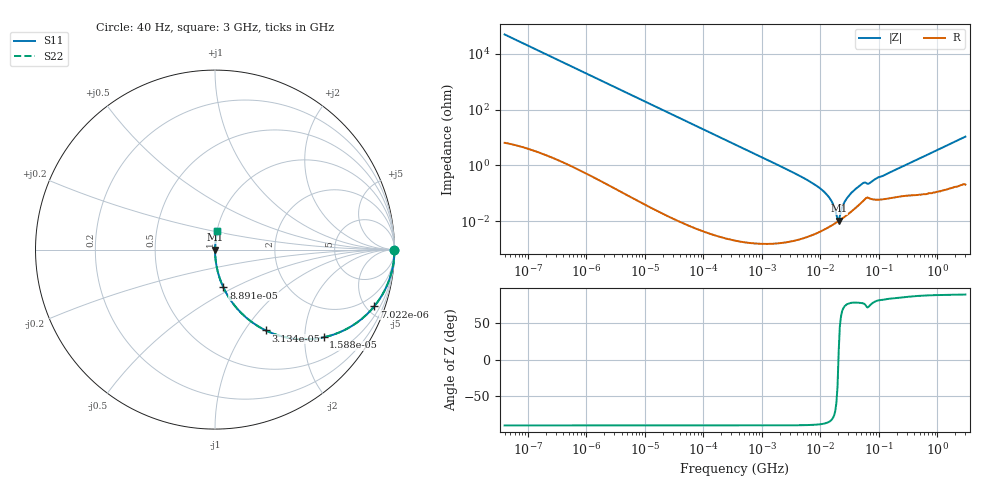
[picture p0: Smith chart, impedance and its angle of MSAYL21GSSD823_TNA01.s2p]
! MSAYL21GSSD823_TNA01  S-PARAMETER MODEL  ( General Type )
! Model Generated by TAIYO YUDEN Corporation (http://www.ty-top.com)
! Version 2.0
! TAIYO YUDEN Control No. 041125
! Copyright(c) 2004 TAIYO YUDEN CO.,LTD. All Rights Reserved.
! Product Description (link to TY-COMPAS)
! https://ds.yuden.co.jp/TYCOMPAS/or/detail?pn=MSAYL21GSSD823KTNA01&u=M
! Products Name : Multilayer Ceramic Capacitors
! Characteristics :
!  Capacitance : 0.082 uF , Rated Voltage : 10V
!  Case Size : 2.0 x 1.25 / 0.079 x 0.049 [mm/inch] , Thickness : 1.25 / 0.049 [mm/inch]
!  (Conditions: Temperature = 25 degC , DC Bias Current/Voltage = 0A / 0V)
! External Node Assignments :
!  1  o---| |---o  2
! GND o---------o GND
! Frequency Range : 40Hz  -  3GHz  [ 401 STEP ]
# MHz S RI R 50
! Freq[MHz].  S11 Real  S11 Imag  S21 Real  S21 Imag  S12 Real  S12 Imag  S22 Real  S22 Imag
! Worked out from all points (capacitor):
!   401 points, 40 Hz to 3 GHz, reference 50 ohm
!   read as one part in series: C = 80.9 nF near 44 Hz
!   lowest |Z| = 10.4 mohm at 20.49 MHz (marker M1)
!   series resonance near 20.3 MHz, so ESL is about 760 pH
!   S11 on the Smith chart (normalised r, x): 40 Hz: open; 7.022 kHz: 1.00, -5.61; 15.88 kHz: 1.00, -2.48; 31.34 kHz: 1.00, -1.26; 88.91 kHz: 1.00, -0.44; 3 GHz: 1.00, +0.22
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4e-05  1 -0.00203  4.4e-06 0.00203  4.4e-06 0.00203  1 -0.00203
0.000834  0.9982 -0.0423  0.0018 0.0423  0.0018 0.0423  0.9982 -0.0423
0.00271  0.9814 -0.1351  0.0186 0.1351  0.0186 0.1351  0.9814 -0.1351
0.007022  0.8871 -0.3164  0.1129 0.3164  0.1129 0.3164  0.8871 -0.3164
0.015879  0.6058 -0.4886  0.3942 0.4886  0.3942 0.4886  0.6058 -0.4886
0.017386  0.5617 -0.4961  0.4383 0.4961  0.4383 0.4961  0.5617 -0.4961
0.031343  0.2829 -0.4503  0.7171 0.4503  0.7171 0.4503  0.2829 -0.4503
0.088912  0.0468 -0.211  0.9532 0.211  0.9532 0.211  0.0468 -0.211
0.362475  0.00296 -0.0541  0.997 0.0541  0.997 0.0541  0.00296 -0.0541
7.222098  3.75e-05 -0.00237  1 0.00237  1 0.00237  3.75e-05 -0.00237
10.37922  4.66e-05 -0.00139  1 0.00139  1 0.00139  4.66e-05 -0.00139
13.62356  6.09e-05 -0.00078  0.9999 0.00078  0.9999 0.00078  6.09e-05 -0.00078
16.33207  7.56e-05 -0.000414  0.9999 0.000414  0.9999 0.000414  7.56e-05 -0.000414
18.71131  9.03e-05 -0.000153  0.9999 0.000153  0.9999 0.000153  9.03e-05 -0.000153
20.48705  0.000102 1.91e-05  0.9999 -1.91e-05  0.9999 -1.91e-05  0.000102 1.91e-05
21.43715  0.000109 0.000111  0.9999 -0.000111  0.9999 -0.000111  0.000109 0.000111
26.8909  0.000154 0.000542  0.9998 -0.000542  0.9998 -0.000542  0.000154 0.000542
38.64618  0.000286 0.00133  0.9997 -0.00133  0.9997 -0.00133  0.000286 0.00133
53.07868  0.000526 0.00225  0.9995 -0.00225  0.9995 -0.00225  0.000526 0.00225
69.67004  0.000659 0.00226  0.9993 -0.00226  0.9993 -0.00226  0.000659 0.00226
150.5692  0.000697 0.00551  0.9993 -0.00551  0.9993 -0.00551  0.000697 0.00551
3000  0.0135 0.1061  0.9865 -0.1061  0.9865 -0.1061  0.0135 0.1061
